(* Logix 5000 Rung export; software revision 16.04; part 2 of 2 *)
(* AOI56PDPMV1_FLEX, continued *)

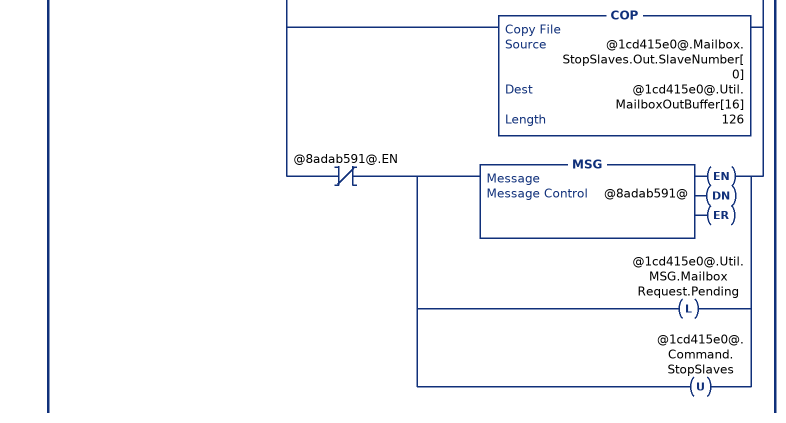
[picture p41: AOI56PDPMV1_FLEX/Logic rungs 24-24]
   // StopSlaves mailbox request.
   // This mailbox allows the interruption of communication to a specific slave
   // This rung initially creates a new mailbox ID by incrementing the last sent mailbox ID by a value of 1.  The mailbox ID is composed of the low byte containing the new mailbox ID and the high byte containing the decimal value of "-20480" (indicating the mailbox from the backplane).
   // This rung will update the MVI56PDPMV1.Util.MailboxOutBuffer according to the specific mailbox request and then execute the MSG instruction.  The MVI56PDPMV1.Util.MSG.MailboxRequest.Pending will be latched until the MSG operation is concluded to prevent other mailbox requests to be performed during that time. If the MSG operation is successfull then the MVI56PDPMV1.Util.MSG.MailboxRequest.DNCounter tag is incremented and the DN bit is cleared. If the MSG is not sucessfull then the MVI56PDPMV1.Util.MSG.MailboxRequest.ERCounter is incremented and the ER bit is cleared. A minimum of 100ms time should be kept between two consecutive requests for better performance, otherwise a MSG error might be returned.
   24: XIC(@1cd415e0@.Command.StopSlaves)XIO(@1cd415e0@.Util.MSG.MailboxRequest.Pending)[[ADD(1,@1cd415e0@.Util.MailboxIDOutLowByte,@1cd415e0@.Util.MailboxIDOutLowByte) ,GEQ(@1cd415e0@.Util.MailboxIDOutLowByte,256) MOV(1,@1cd415e0@.Util.MailboxIDOutLowByte) ,ADD(@1cd415e0@.Util.MailboxIDOutLowByte,-20480,@1cd415e0@.Util.MailboxIDOut) ] ,MOV(@1cd415e0@.Util.MailboxIDOut,@1cd415e0@.Util.MailboxOutBuffer[0]) ,MOV(16386,@1cd415e0@.Util.MailboxOutBuffer[1]) ,MOV(12,@1cd415e0@.Util.MailboxOutBuffer[2]) ,MOV(126,@1cd415e0@.Util.MailboxOutBuffer[3]) ,MOV(1,@1cd415e0@.Util.MailboxOutBuffer[4]) ,MOV(1,@1cd415e0@.Util.MailboxOutBuffer[5]) ,MOV(0,@1cd415e0@.Util.MailboxOutBuffer[6]) ,MOV(0,@1cd415e0@.Util.MailboxOutBuffer[7]) ,MOV(0,@1cd415e0@.Util.MailboxOutBuffer[8]) ,MOV(0,@1cd415e0@.Util.MailboxOutBuffer[9]) ,MOV(0,@1cd415e0@.Util.MailboxOutBuffer[10]) ,MOV(0,@1cd415e0@.Util.MailboxOutBuffer[11]) ,MOV(0,@1cd415e0@.Util.MailboxOutBuffer[12]) ,MOV(0,@1cd415e0@.Util.MailboxOutBuffer[13]) ,MOV(0,@1cd415e0@.Util.MailboxOutBuffer[14]) ,MOV(0,@1cd415e0@.Util.MailboxOutBuffer[15]) ,COP(@1cd415e0@.Mailbox.StopSlaves.Out.SlaveNumber[0],@1cd415e0@.Util.MailboxOutBuffer[16],126) ,XIO(@8adab591@.EN) [MSG(@8adab591@) ,OTL(@1cd415e0@.Util.MSG.MailboxRequest.Pending) ,OTU(@1cd415e0@.Command.StopSlaves) ] ];
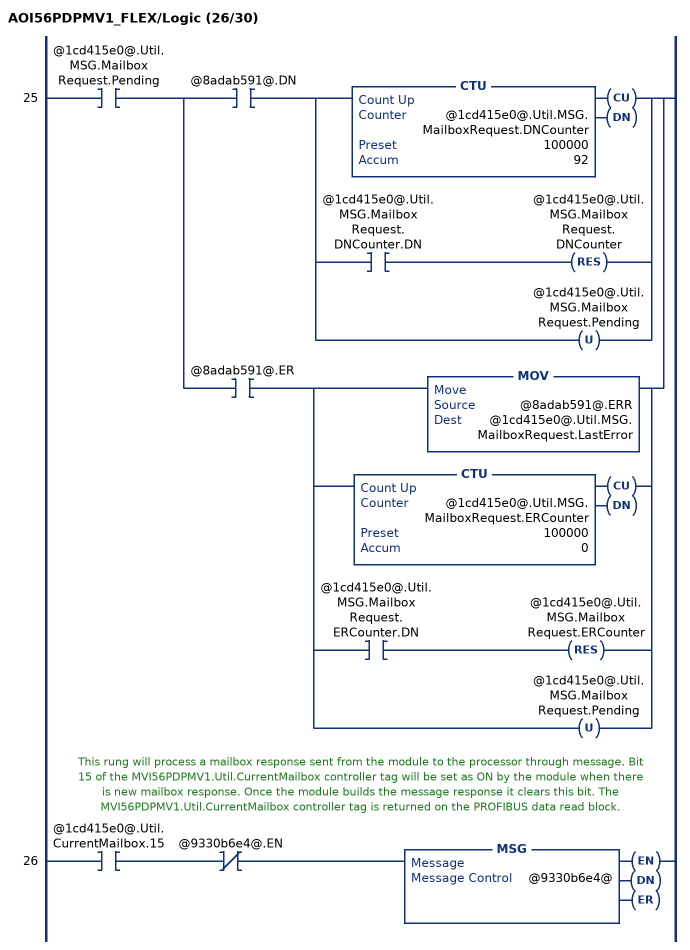
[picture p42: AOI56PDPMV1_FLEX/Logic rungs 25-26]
   25: XIC(@1cd415e0@.Util.MSG.MailboxRequest.Pending)[XIC(@8adab591@.DN) [CTU(@1cd415e0@.Util.MSG.MailboxRequest.DNCounter,100000,92) ,XIC(@1cd415e0@.Util.MSG.MailboxRequest.DNCounter.DN) RES(@1cd415e0@.Util.MSG.MailboxRequest.DNCounter) ,OTU(@1cd415e0@.Util.MSG.MailboxRequest.Pending) ] ,XIC(@8adab591@.ER) [MOV(@8adab591@.ERR,@1cd415e0@.Util.MSG.MailboxRequest.LastError) ,CTU(@1cd415e0@.Util.MSG.MailboxRequest.ERCounter,100000,0) ,XIC(@1cd415e0@.Util.MSG.MailboxRequest.ERCounter.DN) RES(@1cd415e0@.Util.MSG.MailboxRequest.ERCounter) ,OTU(@1cd415e0@.Util.MSG.MailboxRequest.Pending) ] ];
   // This rung will process a mailbox response sent from the module to the processor through message. Bit 15 of the MVI56PDPMV1.Util.CurrentMailbox controller tag will be set as ON by the module when there is new mailbox response. Once the module builds the message response it clears this bit. The  MVI56PDPMV1.Util.CurrentMailbox controller tag is returned on the PROFIBUS data read block.
   26: XIC(@1cd415e0@.Util.CurrentMailbox.15)XIO(@9330b6e4@.EN)MSG(@9330b6e4@);
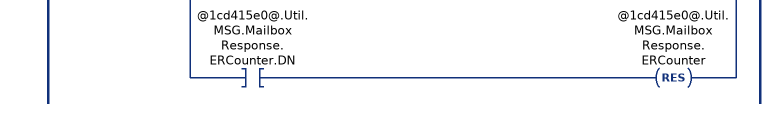
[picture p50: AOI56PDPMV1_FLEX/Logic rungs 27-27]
   // Reads the AcyclicRead mailbox response from the module
   27: [XIC(@9330b6e4@.DN) [EQU(@1cd415e0@.Util.MailboxInBuffer[2],32) [MOV(@1cd415e0@.Util.MailboxInBuffer[3],@1cd415e0@.Mailbox.AcyclicRead.In.ByteCount) ,COP(@1cd415e0@.Util.MailboxInBuffer[8],@1cd415e0@.Mailbox.AcyclicRead.In.SlotNumber,2) ,COP(@1cd415e0@.Util.MailboxInBuffer[9],@1cd415e0@.Mailbox.AcyclicRead.In.Length,2) ,COP(@1cd415e0@.Util.MailboxInBuffer[12],@1cd415e0@.Mailbox.AcyclicRead.In.ErrorDecode,1) ,COP(@1cd415e0@.Util.MailboxInBuffer[13],@1cd415e0@.Mailbox.AcyclicRead.In.ErrorCode2,2) ,MOV(@1cd415e0@.Util.MailboxInBuffer[14],@1cd415e0@.Mailbox.AcyclicRead.In.ExtendedFaultInfo) ,MOV(@1cd415e0@.Util.MailboxInBuffer[15],@1cd415e0@.Mailbox.AcyclicRead.In.FaultInformation) ,COP(@1cd415e0@.Util.MailboxInBuffer[16],@1cd415e0@.Mailbox.AcyclicRead.In.Data[0],@1cd415e0@.Mailbox.AcyclicRead.In.ByteCount) ] ,EQU(@1cd415e0@.Util.MailboxInBuffer[2],33) [MOV(@1cd415e0@.Util.MailboxInBuffer[3],@1cd415e0@.Mailbox.AcyclicWrite.In.ByteCount) ,COP(@1cd415e0@.Util.MailboxInBuffer[8],@1cd415e0@.Mailbox.AcyclicWrite.In.SlotNumber,2) ,COP(@1cd415e0@.Util.MailboxInBuffer[9],@1cd415e0@.Mailbox.AcyclicWrite.In.Length,2) ,COP(@1cd415e0@.Util.MailboxInBuffer[12],@1cd415e0@.Mailbox.AcyclicWrite.In.ErrorDecode,1) ,COP(@1cd415e0@.Util.MailboxInBuffer[13],@1cd415e0@.Mailbox.AcyclicWrite.In.ErrorCode2,2) ,MOV(@1cd415e0@.Util.MailboxInBuffer[14],@1cd415e0@.Mailbox.AcyclicWrite.In.ExtendedFaultInfo) ,MOV(@1cd415e0@.Util.MailboxInBuffer[15],@1cd415e0@.Mailbox.AcyclicWrite.In.FaultInformation) ,COP(@1cd415e0@.Util.MailboxInBuffer[16],@1cd415e0@.Mailbox.AcyclicWrite.In.Data[0],@1cd415e0@.Mailbox.AcyclicWrite.In.ByteCount) ] ,EQU(@1cd415e0@.Util.MailboxInBuffer[2],24) COP(@1cd415e0@.Util.MailboxInBuffer[16],@1cd415e0@.Mailbox.GetLiveList.Station[0],127) ,EQU(@1cd415e0@.Util.MailboxInBuffer[2],5) [MOV(@1cd415e0@.Util.MailboxInBuffer[3],@1cd415e0@.Mailbox.GetSlaveConfig.In.ByteCount) ,MOV(@1cd415e0@.Util.MailboxInBuffer[8],@1cd415e0@.Util.ByteSwapUtil) ,SWPB(@1cd415e0@.Util.ByteSwapUtil,REVERSE,@1cd415e0@.Mailbox.GetSlaveConfig.In.SlaveAddress) ,COP(@1cd415e0@.Util.MailboxInBuffer[12],@1cd415e0@.Mailbox.GetSlaveConfig.In.ErrorCode[0],2) ,MOV(@1cd415e0@.Util.MailboxInBuffer[14],@1cd415e0@.Mailbox.GetSlaveConfig.In.ReturnCode) ,MOV(@1cd415e0@.Util.MailboxInBuffer[15],@1cd415e0@.Mailbox.GetSlaveConfig.In.FaultInformation) ,COP(@1cd415e0@.Util.MailboxInBuffer[16],@1cd415e0@.Mailbox.GetSlaveConfig.In.Identifier[0],@1cd415e0@.Mailbox.GetSlaveConfig.In.ByteCount) ] ,EQU(@1cd415e0@.Util.MailboxInBuffer[2],4) [COP(@1cd415e0@.Util.MailboxInBuffer[8],@1cd415e0@.Mailbox.GetSlaveDiagnostics.In.RequestType,2) ,MOV(@1cd415e0@.Util.MailboxInBuffer[14],@1cd415e0@.Mailbox.GetSlaveDiagnostics.In.ExtendedFaultInfo) ,MOV(@1cd415e0@.Util.MailboxInBuffer[15],@1cd415e0@.Mailbox.GetSlaveDiagnostics.In.FaultInformation) ,MOV(@1cd415e0@.Util.MailboxInBuffer[16],@1cd415e0@.Mailbox.GetSlaveDiagnostics.In.StationStatus1_2) ,MOV(@1cd415e0@.Util.MailboxInBuffer[17],@1cd415e0@.Mailbox.GetSlaveDiagnostics.In.StationStatus3_4) ,MOV(@1cd415e0@.Util.MailboxInBuffer[18],@1cd415e0@.Mailbox.GetSlaveDiagnostics.In.IdentNumber) ,COP(@1cd415e0@.Util.MailboxInBuffer[19],@1cd415e0@.Mailbox.GetSlaveDiagnostics.In.ExtendedDiagnosticData[0],200) ] ,EQU(@1cd415e0@.Util.MailboxInBuffer[2],6) [MOV(@1cd415e0@.Util.MailboxInBuffer[3],@1cd415e0@.Mailbox.SetSlaveAddress.In.ByteCount) ,COP(@1cd415e0@.Util.MailboxInBuffer[8],@1cd415e0@.Mailbox.SetSlaveAddress.In.NewSlaveAddress,2) ,MOV(@1cd415e0@.Util.MailboxInBuffer[9],@1cd415e0@.Mailbox.SetSlaveAddress.In.SlaveIdentNumber) ,MOV(@1cd415e0@.Util.MailboxInBuffer[10],@1cd415e0@.Util.ByteSwapUtil) ,SWPB(@1cd415e0@.Util.ByteSwapUtil,REVERSE,@1cd415e0@.Mailbox.SetSlaveAddress.In.No_add_Chg) ,MOV(@1cd415e0@.Util.MailboxInBuffer[12],@1cd415e0@.Mailbox.SetSlaveAddress.In.ErrorCode1_2) ,MOV(@1cd415e0@.Util.MailboxInBuffer[13],@1cd415e0@.Mailbox.SetSlaveAddress.In.ErrorCode3_4) ,MOV(@1cd415e0@.Util.MailboxInBuffer[14],@1cd415e0@.Mailbox.SetSlaveAddress.In.ReturnCode) ,MOV(@1cd415e0@.Util.MailboxInBuffer[15],@1cd415e0@.Mailbox.SetSlaveAddress.In.FaultInformation) ,COP(@1cd415e0@.Util.MailboxInBuffer[16],@1cd415e0@.Mailbox.SetSlaveAddress.In.MessageDataByte[0],@1cd415e0@.Mailbox.SetSlaveAddress.In.ByteCount) ] ,EQU(@1cd415e0@.Util.MailboxInBuffer[2],3) [COP(@1cd415e0@.Util.MailboxInBuffer[8],@1cd415e0@.Mailbox.SetSlaveMode.In.GroupSelect,2) ,MOV(@1cd415e0@.Util.MailboxInBuffer[9],@1cd415e0@.Util.TempInt) ,SWPB(@1cd415e0@.Util.TempInt,REVERSE,@1cd415e0@.Util.ByteSwapUtil) ,COP(@1cd415e0@.Util.ByteSwapUtil,@1cd415e0@.Mailbox.SetSlaveMode.In.ControlCommand,1) ,MOV(@1cd415e0@.Util.MailboxInBuffer[14],@1cd415e0@.Mailbox.SetSlaveMode.In.ExtendedFaultInfo) ,MOV(@1cd415e0@.Util.MailboxInBuffer[15],@1cd415e0@.Mailbox.SetSlaveMode.In.FaultInformation) ] ,EQU(@1cd415e0@.Util.MailboxInBuffer[2],11) [MOV(@1cd415e0@.Util.MailboxInBuffer[14],@1cd415e0@.Mailbox.StartSlaves.In.AdditionalFaultInfo) ,MOV(@1cd415e0@.Util.MailboxInBuffer[15],@1cd415e0@.Mailbox.StartSlaves.In.FaultInformation) ,COP(@1cd415e0@.Util.MailboxInBuffer[16],@1cd415e0@.Mailbox.StartSlaves.In.SlaveNumber[0],126) ] ,EQU(@1cd415e0@.Util.MailboxInBuffer[2],12) [MOV(@1cd415e0@.Util.MailboxInBuffer[14],@1cd415e0@.Mailbox.StopSlaves.In.AdditionalFaultinfo) ,MOV(@1cd415e0@.Util.MailboxInBuffer[15],@1cd415e0@.Mailbox.StopSlaves.In.FaultInformation) ,COP(@1cd415e0@.Util.MailboxInBuffer[16],@1cd415e0@.Mailbox.StopSlaves.In.SlaveNumber[0],126) ] ,CTU(@1cd415e0@.Util.MSG.MailboxResponse.DNCounter,100000,92) ,XIC(@1cd415e0@.Util.MSG.MailboxResponse.DNCounter.DN) RES(@1cd415e0@.Util.MSG.MailboxResponse.DNCounter) ] ,XIC(@9330b6e4@.ER) [MOV(@9330b6e4@.ERR,@1cd415e0@.Util.MSG.MailboxResponse.LastError) ,CTU(@1cd415e0@.Util.MSG.MailboxResponse.ERCounter,100000,0) ,XIC(@1cd415e0@.Util.MSG.MailboxResponse.ERCounter.DN) RES(@1cd415e0@.Util.MSG.MailboxResponse.ERCounter) ] ];
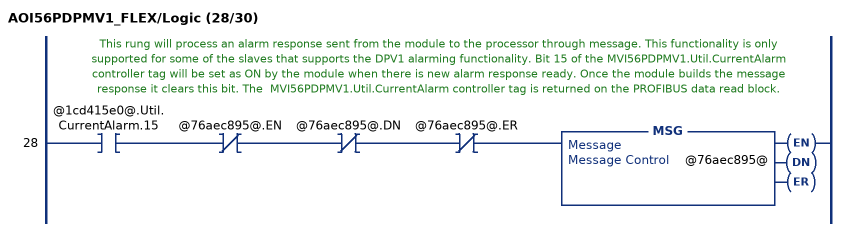
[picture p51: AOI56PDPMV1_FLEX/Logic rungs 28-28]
   // This rung will process an alarm response sent from the module to the processor through message. This functionality is only supported for some of the slaves that supports the DPV1 alarming functionality. Bit 15 of the MVI56PDPMV1.Util.CurrentAlarm controller tag will be set as ON by the module when there is new alarm response ready. Once the module builds the message response it clears this bit. The  MVI56PDPMV1.Util.CurrentAlarm controller tag is returned on the PROFIBUS data read block.
   28: XIC(@1cd415e0@.Util.CurrentAlarm.15)XIO(@76aec895@.EN)XIO(@76aec895@.DN)XIO(@76aec895@.ER)MSG(@76aec895@);
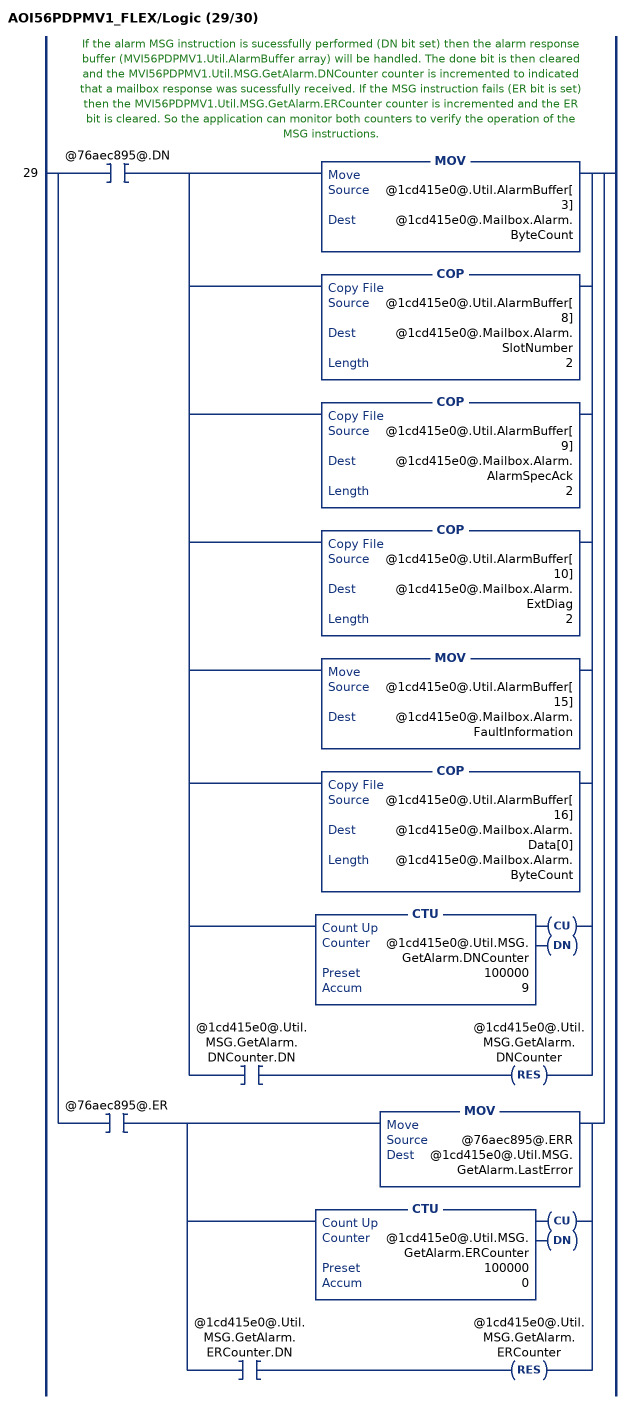
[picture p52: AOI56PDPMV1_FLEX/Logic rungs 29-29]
   // If the alarm MSG instruction is sucessfully performed (DN bit set) then the alarm response buffer (MVI56PDPMV1.Util.AlarmBuffer array) will be handled. The done bit is then cleared and the MVI56PDPMV1.Util.MSG.GetAlarm.DNCounter counter is incremented to indicated that a mailbox response was sucessfully received. If the MSG instruction fails (ER bit is set) then the MVI56PDPMV1.Util.MSG.GetAlarm.ERCounter counter is incremented and the ER bit is cleared. So the application can monitor both counters to verify the operation of the MSG instructions.
   29: [XIC(@76aec895@.DN) [MOV(@1cd415e0@.Util.AlarmBuffer[3],@1cd415e0@.Mailbox.Alarm.ByteCount) ,COP(@1cd415e0@.Util.AlarmBuffer[8],@1cd415e0@.Mailbox.Alarm.SlotNumber,2) ,COP(@1cd415e0@.Util.AlarmBuffer[9],@1cd415e0@.Mailbox.Alarm.AlarmSpecAck,2) ,COP(@1cd415e0@.Util.AlarmBuffer[10],@1cd415e0@.Mailbox.Alarm.ExtDiag,2) ,MOV(@1cd415e0@.Util.AlarmBuffer[15],@1cd415e0@.Mailbox.Alarm.FaultInformation) ,COP(@1cd415e0@.Util.AlarmBuffer[16],@1cd415e0@.Mailbox.Alarm.Data[0],@1cd415e0@.Mailbox.Alarm.ByteCount) ,CTU(@1cd415e0@.Util.MSG.GetAlarm.DNCounter,100000,9) ,XIC(@1cd415e0@.Util.MSG.GetAlarm.DNCounter.DN) RES(@1cd415e0@.Util.MSG.GetAlarm.DNCounter) ] ,XIC(@76aec895@.ER) [MOV(@76aec895@.ERR,@1cd415e0@.Util.MSG.GetAlarm.LastError) ,CTU(@1cd415e0@.Util.MSG.GetAlarm.ERCounter,100000,0) ,XIC(@1cd415e0@.Util.MSG.GetAlarm.ERCounter.DN) RES(@1cd415e0@.Util.MSG.GetAlarm.ERCounter) ] ];
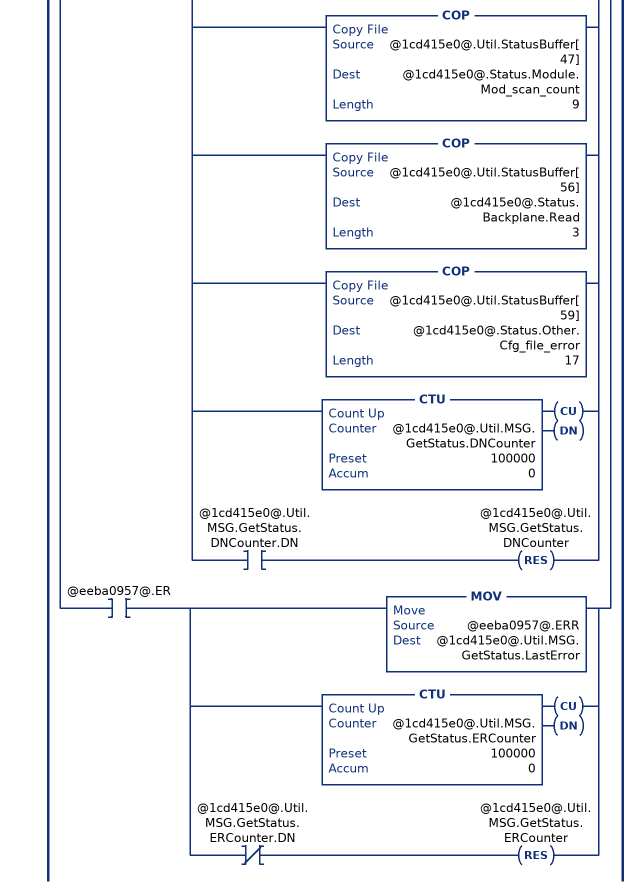
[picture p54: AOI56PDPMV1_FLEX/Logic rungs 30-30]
   // In order to retrieve status information from the module the processor can trigger the MVI56PDPMV1.Command.GetStatus bit that will request the MSG instruction from the module.
   // If the MSG instruction is sucessfully performed (DN bit set) then the status response buffer (MVI56PDPMV1.Util.StatusBuffer array) will be handled. The done bit is then cleared and the MVI56PDPMV1.Util.MSG.GetStatus.DNCounter counter is incremented to indicated that a mailbox response was sucessfully received. If the MSG instruction fails (ER bit is set) then the MVI56PDPMV1.Util.MSG.GetStatus.ERCounter counter is incremented and the ER bit is cleared. So the application can monitor both counters to verify the operation of the MSG instructions.
   // The status information will be copied to the MVI56PDPMV1.Status controller tag
   30: [XIC(@1cd415e0@.Command.GetStatus) XIO(@eeba0957@.EN) [MSG(@eeba0957@) ,OTU(@1cd415e0@.Command.GetStatus) ] ,XIC(@eeba0957@.DN) [COP(@1cd415e0@.Util.StatusBuffer[0],@1cd415e0@.Status.Pattern[0],16) ,COP(@1cd415e0@.Util.StatusBuffer[11],@1cd415e0@.Status.Input_Swap,4) ,COP(@1cd415e0@.Util.StatusBuffer[13],@1cd415e0@.Status.Fieldbus.FB_Slave_Cfg_List[0],52) ,COP(@1cd415e0@.Util.StatusBuffer[39],@1cd415e0@.Status.Control.serial_number[0],8) ,COP(@1cd415e0@.Util.StatusBuffer[43],@1cd415e0@.Status.Profibus_CRC32,2) ,COP(@1cd415e0@.Util.StatusBuffer[47],@1cd415e0@.Status.Module.Mod_scan_count,9) ,COP(@1cd415e0@.Util.StatusBuffer[56],@1cd415e0@.Status.Backplane.Read,3) ,COP(@1cd415e0@.Util.StatusBuffer[59],@1cd415e0@.Status.Other.Cfg_file_error,17) ,CTU(@1cd415e0@.Util.MSG.GetStatus.DNCounter,100000,0) ,XIC(@1cd415e0@.Util.MSG.GetStatus.DNCounter.DN) RES(@1cd415e0@.Util.MSG.GetStatus.DNCounter) ] ,XIC(@eeba0957@.ER) [MOV(@eeba0957@.ERR,@1cd415e0@.Util.MSG.GetStatus.LastError) ,CTU(@1cd415e0@.Util.MSG.GetStatus.ERCounter,100000,0) ,XIO(@1cd415e0@.Util.MSG.GetStatus.ERCounter.DN) RES(@1cd415e0@.Util.MSG.GetStatus.ERCounter) ] ];
END_ROUTINE

ROUTINE Prescan   (* ladder *)
// Power Up Handler
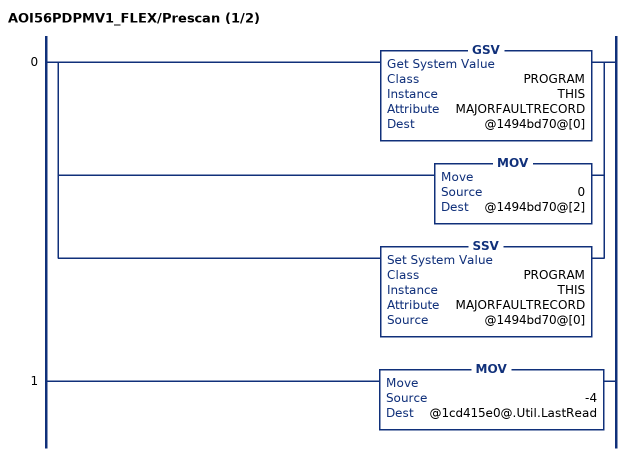
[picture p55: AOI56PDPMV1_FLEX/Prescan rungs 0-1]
   0: [GSV(PROGRAM,THIS,MAJORFAULTRECORD,@1494bd70@[0]) ,MOV(0,@1494bd70@[2]) ,SSV(PROGRAM,THIS,MAJORFAULTRECORD,@1494bd70@[0]) ];
   1: MOV(-4,@1cd415e0@.Util.LastRead);
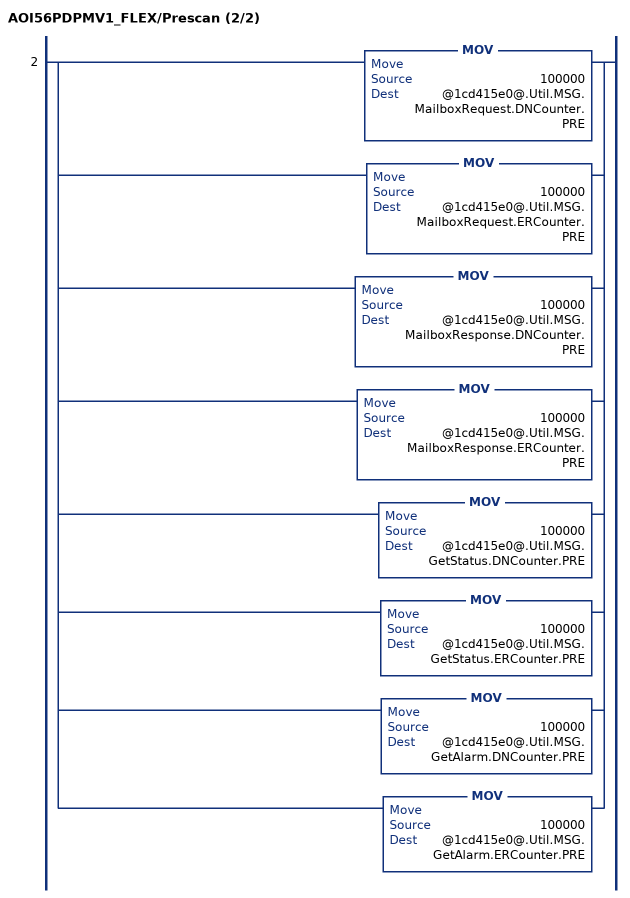
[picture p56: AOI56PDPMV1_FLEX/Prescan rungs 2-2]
   2: [MOV(100000,@1cd415e0@.Util.MSG.MailboxRequest.DNCounter.PRE) ,MOV(100000,@1cd415e0@.Util.MSG.MailboxRequest.ERCounter.PRE) ,MOV(100000,@1cd415e0@.Util.MSG.MailboxResponse.DNCounter.PRE) ,MOV(100000,@1cd415e0@.Util.MSG.MailboxResponse.ERCounter.PRE) ,MOV(100000,@1cd415e0@.Util.MSG.GetStatus.DNCounter.PRE) ,MOV(100000,@1cd415e0@.Util.MSG.GetStatus.ERCounter.PRE) ,MOV(100000,@1cd415e0@.Util.MSG.GetAlarm.DNCounter.PRE) ,MOV(100000,@1cd415e0@.Util.MSG.GetAlarm.ERCounter.PRE) ];
END_ROUTINE
END_ADD_ON_INSTRUCTION

VAR_GLOBAL   (* controller tags *)
   AOI56PDPMV1_FLEX : AOI56PDPMV1_FLEX;
   SetClearMode_MSG : MESSAGE;
        MessageParameters(MessageType := CIP Generic, RequestedLength := 288, ConnectedFlag := 2, ConnectionPath := PDPMV1_FLEX, ServiceCode := 16#0010, ObjectType := 16#0004, TargetObject := 10, AttributeNumber := 16#0001, LocalElement := MVI56PDPMV1.UTIL.MailboxOutBuffer[0])
   GetMailbox_MSG : MESSAGE;
        MessageParameters(MessageType := CIP Generic, ConnectedFlag := 2, ConnectionPath := PDPMV1_FLEX, ServiceCode := 16#000e, ObjectType := 16#0004, TargetObject := 10, AttributeNumber := 16#0001, DestinationTag := MVI56PDPMV1.UTIL.MailboxInBuffer[0])
   GetSlaveCfg_MSG : MESSAGE;
        MessageParameters(MessageType := CIP Generic, RequestedLength := 288, ConnectedFlag := 2, ConnectionPath := PDPMV1_FLEX, ServiceCode := 16#0010, ObjectType := 16#0004, TargetObject := 10, AttributeNumber := 16#0001, LocalElement := MVI56PDPMV1.UTIL.MailboxOutBuffer[0])
   MVI56PDPMV1 : PDPMV1_ModuleDefinition;
   Connection_Input : PDPMV1_Connection_Input;
   SetSlaveAddress_MSG : MESSAGE;
        MessageParameters(MessageType := CIP Generic, RequestedLength := 288, ConnectedFlag := 2, ConnectionPath := PDPMV1_FLEX, ServiceCode := 16#0010, ObjectType := 16#0004, TargetObject := 10, AttributeNumber := 16#0001, LocalElement := MVI56PDPMV1.UTIL.MailboxOutBuffer[0])
   Connection_Output : PDPMV1_Connection_Output;
   SetSlaveMode_MSG : MESSAGE;
        MessageParameters(MessageType := CIP Generic, RequestedLength := 288, ConnectedFlag := 2, ConnectionPath := PDPMV1_FLEX, ServiceCode := 16#0010, ObjectType := 16#0004, TargetObject := 10, AttributeNumber := 16#0001, LocalElement := MVI56PDPMV1.UTIL.MailboxOutBuffer[0])
   GetLiveList_MSG : MESSAGE;
        MessageParameters(MessageType := CIP Generic, RequestedLength := 288, ConnectedFlag := 2, ConnectionPath := PDPMV1_FLEX, ServiceCode := 16#0010, ObjectType := 16#0004, TargetObject := 10, AttributeNumber := 16#0001, LocalElement := MVI56PDPMV1.UTIL.MailboxOutBuffer[0])
   SetOperateMode_MSG : MESSAGE;
        MessageParameters(MessageType := CIP Generic, RequestedLength := 288, ConnectedFlag := 2, ConnectionPath := PDPMV1_FLEX, ServiceCode := 16#0010, ObjectType := 16#0004, TargetObject := 10, AttributeNumber := 16#0001, LocalElement := MVI56PDPMV1.UTIL.MailboxOutBuffer[0])
   GetStatus_MSG : MESSAGE;
        MessageParameters(MessageType := CIP Generic, ConnectedFlag := 2, ConnectionPath := PDPMV1_FLEX, ServiceCode := 16#000e, ObjectType := 16#0004, TargetObject := 9, AttributeNumber := 16#0001, DestinationTag := MVI56PDPMV1.UTIL.StatusBuffer[0])
   StopSlaves_MSG : MESSAGE;
        MessageParameters(MessageType := CIP Generic, RequestedLength := 288, ConnectedFlag := 2, ConnectionPath := PDPMV1_FLEX, ServiceCode := 16#0010, ObjectType := 16#0004, TargetObject := 10, AttributeNumber := 16#0001, LocalElement := MVI56PDPMV1.UTIL.MailboxOutBuffer[0])
   StartSlaves_MSG : MESSAGE;
        MessageParameters(MessageType := CIP Generic, RequestedLength := 288, ConnectedFlag := 2, ConnectionPath := PDPMV1_FLEX, ServiceCode := 16#0010, ObjectType := 16#0004, TargetObject := 10, AttributeNumber := 16#0001, LocalElement := MVI56PDPMV1.UTIL.MailboxOutBuffer[0])
   Local:1:I : AB:1756_MODULE_INT_144Bytes:I:0;
   GetSlaveDiagnostics_MSG : MESSAGE;
        MessageParameters(MessageType := CIP Generic, RequestedLength := 288, ConnectedFlag := 2, ConnectionPath := PDPMV1_FLEX, ServiceCode := 16#0010, ObjectType := 16#0004, TargetObject := 10, AttributeNumber := 16#0001, LocalElement := MVI56PDPMV1.UTIL.MailboxOutBuffer[0])
   SetStopMode_MSG : MESSAGE;
        MessageParameters(MessageType := CIP Generic, RequestedLength := 288, ConnectedFlag := 2, ConnectionPath := PDPMV1_FLEX, ServiceCode := 16#0010, ObjectType := 16#0004, TargetObject := 10, AttributeNumber := 16#0001, LocalElement := MVI56PDPMV1.UTIL.MailboxOutBuffer[0])
   AcyclicWrite_MSG : MESSAGE;
        MessageParameters(MessageType := CIP Generic, RequestedLength := 288, ConnectedFlag := 2, ConnectionPath := PDPMV1_FLEX, ServiceCode := 16#0010, ObjectType := 16#0004, TargetObject := 10, AttributeNumber := 16#0001, LocalElement := MVI56PDPMV1.UTIL.MailboxOutBuffer[0])
   GetAlarm_MSG : MESSAGE;
        MessageParameters(MessageType := CIP Generic, ConnectedFlag := 2, ConnectionPath := PDPMV1_FLEX, ServiceCode := 16#000e, ObjectType := 16#0004, TargetObject := 11, AttributeNumber := 16#0001, DestinationTag := MVI56PDPMV1.UTIL.AlarmBuffer[0])
   AcyclicRead_MSG : MESSAGE;
        MessageParameters(MessageType := CIP Generic, RequestedLength := 288, ConnectedFlag := 2, ConnectionPath := PDPMV1_FLEX, ServiceCode := 16#0010, ObjectType := 16#0004, TargetObject := 10, AttributeNumber := 16#0001, LocalElement := MVI56PDPMV1.UTIL.MailboxOutBuffer[0])
   Local:1:O : AB:1756_MODULE_INT_138Bytes:O:0;
END_VAR

PROGRAM MainProgram

ROUTINE MainRoutine   (* ladder *)
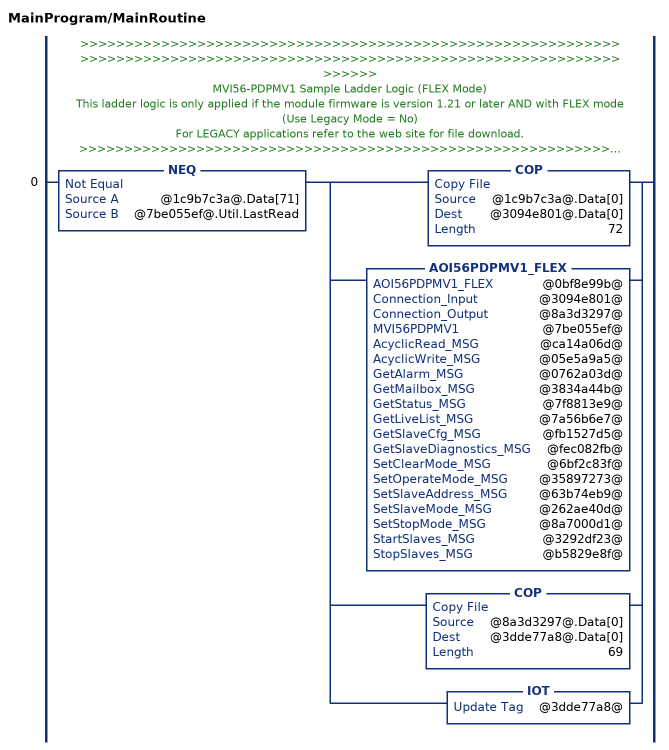
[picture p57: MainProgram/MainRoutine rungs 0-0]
   // >>>>>>>>>>>>>>>>>>>>>>>>>>>>>>>>>>>>>>>>>>>>>>>>>>>>>>>>>>>>>>>>>>>>>>>>>>>>>>>>>>>>>>>>>>>>>>>>>>>>>>>>>>>>>>>>>>>>>>>>>>>>>>
   // MVI56-PDPMV1 Sample Ladder Logic (FLEX Mode)
   // This ladder logic is only applied if the module firmware is version 1.21 or later AND with FLEX mode (Use Legacy Mode = No)
   // For LEGACY applications refer to the web site for file download.
   // >>>>>>>>>>>>>>>>>>>>>>>>>>>>>>>>>>>>>>>>>>>>>>>>>>>>>>>>>>>>>>>>>>>>>>>>>>>>>>>>>>>>>>>>>>>>>>>>>>>>>>>>>>>>>>>>>>>>>>>>>>>>>>>
   // This rung will calculate the sizes of the input and output images configured by the user through RSLogix5000. It also calculates the offset in the read block where  the Read Block ID is located.
   0: NEQ(@1c9b7c3a@.Data[71],@7be055ef@.Util.LastRead)[COP(@1c9b7c3a@.Data[0],@3094e801@.Data[0],72) ,AOI56PDPMV1_FLEX(@0bf8e99b@,@3094e801@,@8a3d3297@,@7be055ef@,@ca14a06d@,@05e5a9a5@,@0762a03d@,@3834a44b@,@7f8813e9@,@7a56b6e7@,@fb1527d5@,@fec082fb@,@6bf2c83f@,@35897273@,@63b74eb9@,@262ae40d@,@8a7000d1@,@3292df23@,@b5829e8f@) ,COP(@8a3d3297@.Data[0],@3dde77a8@.Data[0],69) ,IOT(@3dde77a8@) ];
END_ROUTINE
END_PROGRAM
